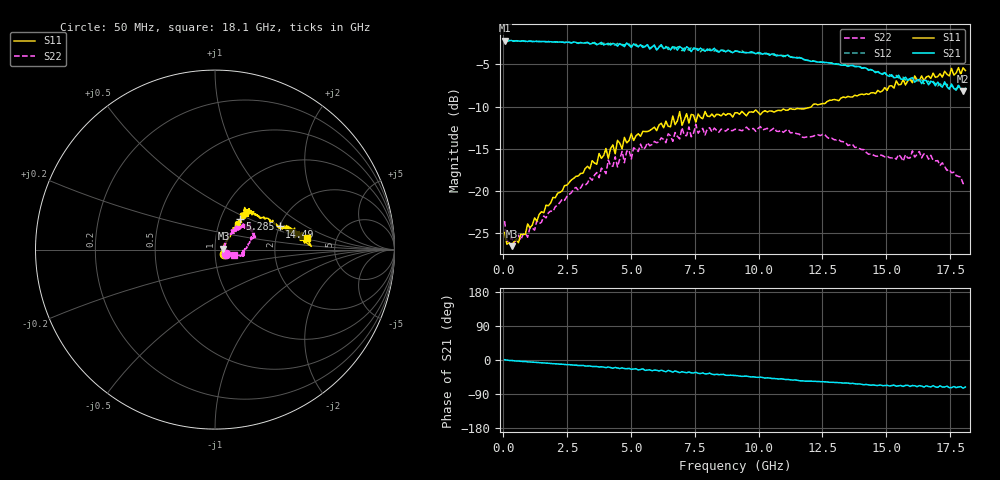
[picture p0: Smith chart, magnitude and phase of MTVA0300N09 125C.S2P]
! Network Analyzer HP8720D.06.14 Serial No. US36140669
! 28 Jun 2005  09:35:10
! Frequency  S11  S21  S12  S22
# HZ  S  DB R 50
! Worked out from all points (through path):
!   201 points, 50 MHz to 18.1 GHz, reference 50 ohm
!   highest |S21| = -2.16 dB at 50 MHz (marker M1); lowest = -8.1 dB at 18.01 GHz (marker M2)
!   group delay of S21, straight-line fit = 11.7 ps
!   lowest |S11| = -26.6 dB at 320.8 MHz (marker M3), VSWR 1.10, Z = 54.9 + j0.555 ohm
!   |S11| at or under -10 dB: start of sweep to 12.07 GHz
!   |S22| runs from -26.2 to -12.1 dB; largest |S21 - S12| = 0.047
!   S11 on the Smith chart (normalised r, x): 50 MHz: 1.11, -0.05; 5.285 GHz: 1.24, +0.44; 14.49 GHz: 2.00, +0.61; 18.1 GHz: 3.04, +0.52
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5e7  -24.93 -23.7  -2.16 0.7  -2.19 0.7  -23.58 -22.1
1.4025e8  -26.33 -10.0  -2.28 -0.3  -2.27 -0.4  -25.96 -8.9
3.2075e8  -26.55 6.2  -2.16 -1.1  -2.20 -1.1  -25.54 3.0
9.525e8  -23.91 25.7  -2.28 -4.9  -2.21 -4.8  -25.50 22.7
3.1185e9  -17.91 44.8  -2.46 -14.2  -2.50 -14.7  -19.20 45.3
4.47225e9  -14.01 44.2  -2.82 -21.1  -2.50 -20.6  -17.17 49.3
4.65275e9  -15.00 44.5  -2.71 -20.8  -2.63 -23.0  -15.32 48.7
5.2845e9  -13.22 50.5  -2.90 -26.3  -2.91 -25.1  -15.33 40.1
6.09675e9  -12.19 48.1  -2.99 -29.0  -2.87 -28.8  -14.19 40.4
6.7285e9  -12.14 54.5  -2.96 -28.9  -3.31 -29.3  -13.08 35.7
6.909e9  -10.60 50.2  -2.88 -33.4  -2.88 -31.2  -13.83 36.0
6.99925e9  -12.22 50.9  -3.07 -30.8  -3.38 -33.0  -12.51 36.6
7.36025e9  -10.93 45.4  -3.48 -34.0  -3.02 -33.7  -13.57 39.0
7.54075e9  -11.85 48.2  -3.12 -32.2  -3.12 -36.0  -12.12 37.1
9.075e9  -10.73 47.7  -3.43 -41.1  -3.40 -41.4  -12.68 24.9
1.21435e10  -9.73 33.5  -4.61 -56.1  -4.57 -56.3  -13.52 19.6
1.449e10  -8.35 19.8  -5.74 -65.7  -5.76 -66.3  -15.74 0.9
1.512175e10  -7.55 15.7  -6.43 -68.6  -6.20 -68.3  -16.06 -3.1
1.674625e10  -6.66 8.9  -6.99 -71.1  -7.36 -70.9  -15.79 -13.1
1.782925e10  -5.38 9.2  -7.41 -71.1  -7.67 -70.9  -18.28 -14.7
1.800975e10  -5.40 1.9  -8.14 -74.4  -7.95 -73.9  -19.14 -10.0
1.81e10  -5.73 6.9  -7.83 -71.3  -8.12 -71.8  -18.97 -16.3
